| IBIS file stm32n657_vfbga169.ibs
[IBIS ver] 4.2
[File name] stm32n657_vfbga169.ibs
[File Rev] 1.1
[Date] 20-09-2024
[Source] Data Created at STMicroelectronics
[Notes]  File originated from ELDO simulations.
[Disclaimer]  This information is for modeling purpose only and is
   not guaranteed. The information is subject to change without
   notice.
[Copyright] Copyright 2024 STMicroelectronics Inc.
|   Component stm32n657_vfbga169
[Component] stm32n657_vfbga169
[Manufacturer] STMicroelectronics
[Package]
| variable   typ   min   max
R_pkg  0  NA  NA
L_pkg  0  NA  NA
C_pkg  0  NA  NA
[Pin]   signal_name   model_name
A1  PDR_ON  nc
A2  NC  nc
A3  OTG2_HSDM  USB2_HS_IBIS
A4  NC  nc
A5  OTG1_HSDM  USB2_HS_IBIS
A6  OTG1_TXRTUNE  nc
A7  PH1-OSC_OUT  isudq_tt
A8  PC11  io8_tt_i3c
A9  PE11  io8_tt
A10  PE13  io8_tt_i3c
A11  PD7  io8_tt
A12  PD1  io8_tt
A13  VSS  gnd
B1  PC14-OSC32_IN  io8_tt_sw
B2  OTG2_ID  nc
B3  OTG2_HSDP  USB2_HS_IBIS
B4  OTG1_ID  nc
B5  OTG1_HSDP  USB2_HS_IBIS
B6  UCPD1_CC1  nc
B7  PH0-OSC_IN  isudq_tt
B8  PC12  io8_tt
B9  PE14  io8_tt_i3c
B10  PE12  io8_tt
B11  PD10  io8_tt
B12  PD0  io8_tt
B13  PD15  io8_tt_i3c
C1  PC15-OSC32_OUT  io8_tt_sw
C2  VBAT  power
C3  OTG2_TXRTUNE  nc
C4  VDDA18USB  power
C5  VDD33USB  power
C6  UCPD1_CC2  nc
C7  PC9  io8_tt_i3c
C8  PH2  io8_tt
C9  PE5  io8_tt_i3c
C10  PD2  io8_tt
C11  PE7  io8_tt
C12  PD3  io8_tt_i3c
C13  PD14  io8_tt_i3c
D1  V08CAP  nc
D2  PC13  io8_tt_tamp
D3  BOOT0  isudq_tt
D4  PWR_ON  io8_tt
D5  VDDA18AON  nc
D6  PC10  io8_tt_i3c
D7  PC8  io8_tt_i3c
D8  VDDIO4  power
D9  PE15  io8_tt_i3c
D10  PD6  io8_tt
D11  PD12  io8_tt
D12  PE8  io8_tt
D13  PD4  io8_tt_i3c
E1  VDDA18PMU  nc
E2  VSSAPMU  nc
E3  VFBSMPS  nc
E4  NRST  ioreset_tt_v18_1v8
E5  VSSAON  nc
E6  VSS  gnd
E7  VDDCORE  nc
E8  VSS  gnd
E9  VDD  power
E10  PB3  io8_tt
E11  PD8  io8_tt
E12  PE10  io8_tt
E13  PE9  io8_tt
F1  VSSSMPS  nc
F2  VSSSMPS  nc
F3  VSSSMPS  nc
F4  VSSSMPS  nc
F5  VSS  gnd
F6  VDDCORE  nc
F7  VSS  gnd
F8  VDDCORE  nc
F9  VSS  gnd
F10  PE2  io8_tt
F11  PE1  io8_tt
F12  PE0  io8_tt
F13  PD11  io8_tt_i3c
G1  VLXSMPS  nc
G2  VLXSMPS  nc
G3  VLXSMPS  nc
G4  VLXSMPS  nc
G5  VDDCORE  nc
G6  VSS  gnd
G7  VDDCORE  nc
G8  VSS  gnd
G9  VDD  power
G10  PB7  io8_tt
G11  PB6  io8_tt
G12  PB0  io8_tt
G13  PE3  io8_tt
H1  VDDSMPS  nc
H2  VDDSMPS  nc
H3  VDDSMPS  nc
H4  VDDSMPS  nc
H5  VSS  gnd
H6  VDDCORE  nc
H7  VSS  gnd
H8  VDDCORE  nc
H9  VSS  gnd
H10  VDDIO3  power
H11  PN11  io8_tt
H12  PN3  io8_tt
H13  PN1  io8_tt
J1  PF4  io8_tt
J2  PF10  io8_tt
J3  PF5  io8_tt
J4  PF3  io8_tt
J5  VDDA18PLL  nc
J6  VSS  gnd
J7  VDDCORE  nc
J8  VSS  gnd
J9  VDD  power
J10  VDDIO3  power
J11  PN2  io8_tt
J12  PN10  io8_tt
J13  PN0  io8_tt
K1  PF2  io8_tt
K2  PF14  io8_tt
K3  PF15  io8_tt
K4  PF7  io8_tt
K5  VSSA  nc
K6  PG14  io8_tt
K7  PA12  io8_tt
K8  PA2  io8_tt
K9  PG13  io8_tt
K10  PB12  io8_tt_i3c
K11  PN7  io8_tt
K12  PN6  io8_tt
K13  PN9  io8_tt
L1  PF8  io8_tt
L2  PF11  io8_tt
L3  PF12  io8_tt
L4  PF13  io8_tt
L5  VDDA18ADC  nc
L6  VDDCSI  nc
L7  PA11  io8_tt
L8  PA8  io8_tt_i3c
L9  PA1  io8_tt
L10  PB11  io8_tt_i3c
L11  PB5  io8_tt_i3c
L12  PN4  io8_tt
L13  PN5  io8_tt
M1  VREFP  nc
M2  CSI_D1N  DPHY_IBIS_L1
M3  CSI_CKN  DPHY_IBIS_L1
M4  CSI_D0N  DPHY_IBIS_L1
M5  VDDA18CSI  power
M6  PA13  io8_tt
M7  PA9  io8_tt_i3c
M8  PA5  io8_tt_i3c
M9  PA0  io8_tt
M10  PB10  io8_tt_i3c
M11  PB4  io8_tt
M12  PN12  io8_tt
M13  PN8  io8_tt
N1  VSS  gnd
N2  CSI_D1P  DPHY_IBIS_L1
N3  CSI_CKP  DPHY_IBIS_L1
N4  CSI_D0P  DPHY_IBIS_L1
N5  CSI_REXT  nc
N6  PA14  io8_tt
N7  PA10  io8_tt
N8  PA6  io8_tt_i3c
N9  PG10  io8_tt
N10  PG2  io8_tt
N11  PA15  io8_tt
N12  PA3  io8_tt
N13  VSS  gnd
[Package Model]   486-fcvfbga-6x6-169-240308
[Pin Mapping]   pulldown_ref   pullup_ref   | Comment
A1  nc  nc
A2  nc  nc
A3  gnd  VDD33USB
A4  nc  nc
A5  gnd  VDD33USB
A6  nc  nc
A7  gnd  VDD
A8  gnd  VDDIO4
A9  gnd  VDD
A10  gnd  VDD
A11  gnd  VDD
A12  gnd  VDD
A13  gnd  nc
B1  gnd  VSW
B2  nc  nc
B3  gnd  VDD33USB
B4  nc  nc
B5  gnd  VDD33USB
B6  nc  nc
B7  gnd  VDD
B8  gnd  VDDIO4
B9  gnd  VDD
B10  gnd  VDD
B11  gnd  VDD
B12  gnd  VDD
B13  gnd  VDD
C1  gnd  VSW
C2  nc  VSW
C3  nc  nc
C4  nc  VDDA18USB
C5  nc  VDD33USB
C6  nc  nc
C7  gnd  VDDIO4
C8  gnd  VDDIO4
C9  gnd  VDD
C10  gnd  VDD
C11  gnd  VDD
C12  gnd  VDD
C13  gnd  VDD
D1  nc  nc
D2  gnd  VSW
D3  gnd  VDD
D4  gnd  VDD
D5  nc  nc
D6  gnd  VDDIO4
D7  gnd  VDDIO4
D8  nc  VDDIO4
D9  gnd  VDD
D10  gnd  VDD
D11  gnd  VDD
D12  gnd  VDD
D13  gnd  VDD
E1  nc  nc
E2  nc  nc
E3  nc  nc
E4  gnd  VDD
E5  nc  nc
E6  gnd  nc
E7  nc  nc
E8  gnd  nc
E9  nc  VDD
E10  gnd  VDD
E11  gnd  VDD
E12  gnd  VDD
E13  gnd  VDD
F1  nc  nc
F2  nc  nc
F3  nc  nc
F4  nc  nc
F5  gnd  nc
F6  nc  nc
F7  gnd  nc
F8  nc  nc
F9  gnd  nc
F10  gnd  VDD
F11  gnd  VDD
F12  gnd  VDD
F13  gnd  VDD
G1  nc  nc
G2  nc  nc
G3  nc  nc
G4  nc  nc
G5  nc  nc
G6  gnd  nc
G7  nc  nc
G8  gnd  nc
G9  nc  VDD
G10  gnd  VDD
G11  gnd  VDD
G12  gnd  VDD
G13  gnd  VDD
H1  nc  nc
H2  nc  nc
H3  nc  nc
H4  nc  nc
H5  gnd  nc
H6  nc  nc
H7  gnd  nc
H8  nc  nc
H9  gnd  nc
H10  nc  VDDIO3
H11  gnd  VDDIO3
H12  gnd  VDDIO3
H13  gnd  VDDIO3
J1  gnd  VDD
J2  gnd  VDD
J3  gnd  VDD
J4  gnd  VDD
J5  nc  nc
J6  gnd  nc
J7  nc  nc
J8  gnd  nc
J9  nc  VDD
J10  nc  VDDIO3
J11  gnd  VDDIO3
J12  gnd  VDDIO3
J13  gnd  VDDIO3
K1  gnd  VDD
K2  gnd  VDD
K3  gnd  VDD
K4  gnd  VDD
K5  nc  nc
K6  gnd  VDD
K7  gnd  VDD
K8  gnd  VDD
K9  gnd  VDD
K10  gnd  VDD
K11  gnd  VDDIO3
K12  gnd  VDDIO3
K13  gnd  VDDIO3
L1  gnd  VDD
L2  gnd  VDD
L3  gnd  VDD
L4  gnd  VDD
L5  nc  nc
L6  nc  nc
L7  gnd  VDD
L8  gnd  VDD
L9  gnd  VDD
L10  gnd  VDD
L11  gnd  VDD
L12  gnd  VDDIO3
L13  gnd  VDDIO3
M1  nc  nc
M2  gnd  VDDA18CSI
M3  gnd  VDDA18CSI
M4  gnd  VDDA18CSI
M5  nc  VDDA18CSI
M6  gnd  VDD
M7  gnd  VDD
M8  gnd  VDD
M9  gnd  VDD
M10  gnd  VDD
M11  gnd  VDD
M12  gnd  VDDIO3
M13  gnd  VDDIO3
N1  gnd  nc
N2  gnd  VDDA18CSI
N3  gnd  VDDA18CSI
N4  gnd  VDDA18CSI
N5  nc  nc
N6  gnd  VDD
N7  gnd  VDD
N8  gnd  VDD
N9  gnd  VDD
N10  gnd  VDD
N11  gnd  VDD
N12  gnd  VDD
N13  gnd  nc
[Diff Pin]  inv_pin  vdiff  tdelay_typ  tdelay_min  tdelay_max
N3  M3  NA  NA  NA  NA
N4  M4  NA  NA  NA  NA
N2  M2  NA  NA  NA  NA
B5  A5  NA  NA  NA  NA
B3  A3  NA  NA  NA  NA
[Model Selector] DPHY_IBIS_L1
DPHY_RX_2P5G_L1   DPHY HSRX model at 2.5Gbps for lane 1
DPHY_RX_1P5G_L1   DPHY HSRX model at 1.5Gbps for lane 1
[Model Selector] io8_tt
io8_tt_ls_3v3 "GPIO - 3V tolerant - low speed - 3.3V range"
io8_tt_ms_3v3 "GPIO - 3V tolerant - med speed - 3.3V range"
io8_tt_fs_3v3 "GPIO - 3V tolerant - fast speed - 3.3V range"
io8_tt_hs_3v3 "GPIO - 3V tolerant - high speed - 3.3V range"
io8_tt_hslv_ls_1v8 "GPIO low voltage optimization - 3V tolerant - low speed - 1.8V range"
io8_tt_hslv_ms_1v8 "GPIO low voltage optimization - 3V tolerant - med speed - 1.8V range"
io8_tt_hslv_fs_1v8 "GPIO low voltage optimization - 3V tolerant - fast speed - 1.8V range"
io8_tt_hslv_hs_1v8 "GPIO low voltage optimization - 3V tolerant - high speed - 1.8V range"
[Model Selector] io8_tt_i3c
io8_tt_ls_3v3 "GPIO - 3V tolerant - low speed - 3.3V range"
io8_tt_ms_3v3 "GPIO - 3V tolerant - med speed - 3.3V range"
io8_tt_fs_3v3 "GPIO - 3V tolerant - fast speed - 3.3V range"
io8_tt_hs_3v3 "GPIO - 3V tolerant - high speed - 3.3V range"
io8_tt_hslv_ls_1v8 "GPIO low voltage optimization - 3V tolerant - low speed - 1.8V range"
io8_tt_hslv_ms_1v8 "GPIO low voltage optimization - 3V tolerant - med speed - 1.8V range"
io8_tt_hslv_fs_1v8 "GPIO low voltage optimization - 3V tolerant - fast speed - 1.8V range"
io8_tt_hslv_hs_1v8 "GPIO low voltage optimization - 3V tolerant - high speed - 1.8V range"
io8_tt_i3c_ls_3v3 "GPIO with I3C open-drain - 3V tolerant - low speed - 3.3V range"
io8_tt_i3c_ms_3v3 "GPIO with I3C open-drain - 3V tolerant - med speed - 3.3V range"
io8_tt_i3c_fs_3v3 "GPIO with I3C open-drain - 3V tolerant - fast speed - 3.3V range"
io8_tt_i3c_hs_3v3 "GPIO with I3C open-drain - 3V tolerant - high speed - 3.3V range"
io8_tt_hslv_i3c_ls_1v8 "GPIO low voltage optimization with I3C open-drain - 3V tolerant - low speed - 1.8V range"
io8_tt_hslv_i3c_ms_1v8 "GPIO low voltage optimization with I3C open-drain - 3V tolerant - med speed - 1.8V range"
io8_tt_hslv_i3c_fs_1v8 "GPIO low voltage optimization with I3C open-drain - 3V tolerant - fast speed - 1.8V range"
io8_tt_hslv_i3c_hs_1v8 "GPIO low voltage optimization with I3C open-drain - 3V tolerant - high speed - 1.8V range"
io8_tt_i3c_fmp_3v3 "GPIO with I3C fm+ open-drain - 3V tolerant - 3.3V range"
[Model Selector] io8_tt_sw
io8_tt_sw_3v3 "Input Buffer - 3V tolerant - 3.3V range"
io8_tt_sw_1v8 "Input Buffer - 3V tolerant - 1.8V range"
[Model Selector] io8_tt_tamp
io8_tt_ls_3v3 "GPIO - 3V tolerant - low speed - 3.3V range"
io8_tt_ms_3v3 "GPIO - 3V tolerant - med speed - 3.3V range"
io8_tt_fs_3v3 "GPIO - 3V tolerant - fast speed - 3.3V range"
io8_tt_hs_3v3 "GPIO - 3V tolerant - high speed - 3.3V range"
io8_tt_hslv_ls_1v8 "GPIO low voltage optimization - 3V tolerant - low speed - 1.8V range"
io8_tt_hslv_ms_1v8 "GPIO low voltage optimization - 3V tolerant - med speed - 1.8V range"
io8_tt_hslv_fs_1v8 "GPIO low voltage optimization - 3V tolerant - fast speed - 1.8V range"
io8_tt_hslv_hs_1v8 "GPIO low voltage optimization - 3V tolerant - high speed - 1.8V range"
io8_tt_tamp_3v3 "IO tamper - 3V tolerant - 3.3V range"
io8_tt_tamp_1v8 "IO tamper - 3V tolerant - 1.8V range"
|[Model Selector] ioreset_tt_v18
|ioreset_tt_v18_1v8 "Reset PAD - 3V tolerant - 1.8V range"
[Model Selector] isudq_tt
isudq_tt_3v3 "Input Buffer - 3V tolerant - 3.3V range"
isudq_tt_1v8 "Input Buffer - 3V tolerant - 1.8V range"
[Model Selector] USB2_HS_IBIS
USB2_HSRX   USB2 HSRX model
USB2_HSTX_00_0_01_0011_11   TuningBits_AMP_PULSE_RISE_REF_XV=00_0_01_0011_11
USB2_HSTX_00_0_10_0101_11   TuningBits_AMP_PULSE_RISE_REF_XV=00_0_10_0101_11
USB2_HSTX_00_0_11_0111_11   TuningBits_AMP_PULSE_RISE_REF_XV=00_0_11_0111_11
USB2_HSTX_00_1_01_0011_11   TuningBits_AMP_PULSE_RISE_REF_XV=00_1_01_0011_11
USB2_HSTX_00_1_10_0101_11   TuningBits_AMP_PULSE_RISE_REF_XV=00_1_10_0101_11
USB2_HSTX_00_1_11_0111_11   TuningBits_AMP_PULSE_RISE_REF_XV=00_1_11_0111_11
USB2_HSTX_01_0_01_0011_11   TuningBits_AMP_PULSE_RISE_REF_XV=01_0_01_0011_11
USB2_HSTX_01_0_10_0101_11   TuningBits_AMP_PULSE_RISE_REF_XV=01_0_10_0101_11
USB2_HSTX_01_0_11_0111_11   TuningBits_AMP_PULSE_RISE_REF_XV=01_0_11_0111_11
USB2_HSTX_01_1_01_0011_11   TuningBits_AMP_PULSE_RISE_REF_XV=01_1_01_0011_11
USB2_HSTX_01_1_10_0101_11   TuningBits_AMP_PULSE_RISE_REF_XV=01_1_10_0101_11
USB2_HSTX_01_1_11_0111_11   TuningBits_AMP_PULSE_RISE_REF_XV=01_1_11_0111_11
USB2_HSTX_10_0_01_0011_11   TuningBits_AMP_PULSE_RISE_REF_XV=10_0_01_0011_11
USB2_HSTX_10_0_10_0101_11   TuningBits_AMP_PULSE_RISE_REF_XV=10_0_10_0101_11
USB2_HSTX_10_0_11_0111_11   TuningBits_AMP_PULSE_RISE_REF_XV=10_0_11_0111_11
USB2_HSTX_10_1_01_0011_11   TuningBits_AMP_PULSE_RISE_REF_XV=10_1_01_0011_11
USB2_HSTX_10_1_10_0101_11   TuningBits_AMP_PULSE_RISE_REF_XV=10_1_10_0101_11
USB2_HSTX_10_1_11_0111_11   TuningBits_AMP_PULSE_RISE_REF_XV=10_1_11_0111_11
[Define Package Model]  486-fcvfbga-6x6-169-240308
[Manufacturer]  unknown
[OEM]  unknown
[Description]  unknown
[Number Of Pins]  136
[Pin Numbers]
| Pin Name Terminal   Net Name   Starting Node   Ending Node
D3 | BOOT0
M3 | CSI_CKN
N3 | CSI_CKP
M4 | CSI_D0N
N4 | CSI_D0P
M2 | CSI_D1N
N2 | CSI_D1P
N5 | CSI_REXT
E4 | NRST
A5 | OTG1_HSDM
B5 | OTG1_HSDP
B4 | OTG1_ID
A6 | OTG1_TXRTUNE
A4 | NC
A3 | OTG2_HSDM
B3 | OTG2_HSDP
B2 | OTG2_ID
C3 | OTG2_TXRTUNE
A2 | NC
M9 | PA0
L9 | PA1
K8 | PA2
N12 | PA3
M8 | PA5
N8 | PA6
L8 | PA8
M7 | PA9
N7 | PA10
L7 | PA11
K7 | PA12
M6 | PA13
N6 | PA14
N11 | PA15
G12 | PB0
E10 | PB3
M11 | PB4
L11 | PB5
G11 | PB6
G10 | PB7
M10 | PB10
L10 | PB11
K10 | PB12
D7 | PC8
C7 | PC9
D6 | PC10
A8 | PC11
B8 | PC12
D2 | PC13
B1 | PC14-OSC32_IN
C1 | PC15-OSC32_OUT
B12 | PD0
A12 | PD1
C10 | PD2
C12 | PD3
D13 | PD4
D10 | PD6
A11 | PD7
E11 | PD8
B11 | PD10
F13 | PD11
D11 | PD12
C13 | PD14
B13 | PD15
A1 | PDR_ON
F12 | PE0
F11 | PE1
F10 | PE2
G13 | PE3
C9 | PE5
C11 | PE7
D12 | PE8
E13 | PE9
E12 | PE10
A9 | PE11
B10 | PE12
A10 | PE13
B9 | PE14
D9 | PE15
K1 | PF2
J4 | PF3
J1 | PF4
J3 | PF5
K4 | PF7
L1 | PF8
J2 | PF10
L2 | PF11
L3 | PF12
L4 | PF13
K2 | PF14
K3 | PF15
N10 | PG2
N9 | PG10
K9 | PG13
K6 | PG14
B7 | PH0-OSC_IN
A7 | PH1-OSC_OUT
C8 | PH2
J13 | PN0
H13 | PN1
J11 | PN2
H12 | PN3
L12 | PN4
L13 | PN5
K12 | PN6
K11 | PN7
M13 | PN8
K13 | PN9
J12 | PN10
H11 | PN11
M12 | PN12
D4 | PWR_ON
B6 | UCPD1_CC1
C6 | UCPD1_CC2
D1 | V08CAP
C2 | VBAT
C5 | VDD33USB
E9 | VDD
L5 | VDDA18ADC
D5 | VDDA18AON
M5 | VDDA18CSI
J5 | VDDA18PLL
E1 | VDDA18PMU
C4 | VDDA18USB
E7 | VDDCORE
L6 | VDDCSI
H10 | VDDIO3
D8 | VDDIO4
H1 | VDDSMPS
E3 | VFBSMPS
G1 | VLXSMPS
M1 | VREFP
A13 | VSS
K5 | VSSA
E5 | VSSAON
E2 | VSSAPMU
F1 | VSSSMPS
|[Merged Pins]  E9
|G9  |  VDD
|J9  |  VDD
|[Merged Pins]  E7
|F6  |  VDDCORE
|F8  |  VDDCORE
|G5  |  VDDCORE
|G7  |  VDDCORE
|H6  |  VDDCORE
|H8  |  VDDCORE
|J7  |  VDDCORE
|[Merged Pins]  H10
|J10  |  VDDIO3
|[Merged Pins]  H1
|H2  |  VDDSMPS
|H3  |  VDDSMPS
|H4  |  VDDSMPS
|[Merged Pins]  G1
|G2  |  VLXSMPS
|G3  |  VLXSMPS
|G4  |  VLXSMPS
|[Merged Pins]  A13
|E6  |  VSS
|E8  |  VSS
|F5  |  VSS
|F7  |  VSS
|F9  |  VSS
|G6  |  VSS
|G8  |  VSS
|H5  |  VSS
|H7  |  VSS
|H9  |  VSS
|J6  |  VSS
|J8  |  VSS
|N1  |  VSS
|N13  |  VSS
|[Merged Pins]  F1
|F2  |  VSSSMPS
|F3  |  VSSSMPS
|F4  |  VSSSMPS
[Model Data]
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[End Model Data]
[End Package Model]
|End [Component]
| Models and submodels in the file (45): DPHY_RX_1P5G_L1 (Input), DPHY_RX_2P5G_L1 (Input), io8_tt_fs_3v3 (I/O), io8_tt_hs_3v3 (I/O), io8_tt_hslv_fs_1v8 (I/O), io8_tt_hslv_hs_1v8 (I/O), io8_tt_hslv_i3c_fs_1v8 (I/O_open_drain), io8_tt_hslv_i3c_hs_1v8 (I/O_open_drain), io8_tt_hslv_i3c_ls_1v8 (I/O_open_drain), io8_tt_hslv_i3c_ms_1v8 (I/O_open_drain), io8_tt_hslv_ls_1v8 (I/O), io8_tt_hslv_ms_1v8 (I/O), io8_tt_i3c_fmp_3v3 (I/O_open_drain), io8_tt_i3c_fs_3v3 (I/O_open_drain), io8_tt_i3c_hs_3v3 (I/O_open_drain), io8_tt_i3c_ls_3v3 (I/O_open_drain), io8_tt_i3c_ms_3v3 (I/O_open_drain), io8_tt_ls_3v3 (I/O), io8_tt_ms_3v3 (I/O), io8_tt_sw_1v8 (I/O), io8_tt_sw_3v3 (I/O), io8_tt_tamp_1v8 (I/O), io8_tt_tamp_3v3 (I/O), ioreset_tt_v18_1v8 (I/O_open_drain), isudq_tt_1v8 (Input), isudq_tt_3v3 (Input), USB2_HSRX (Input), USB2_HSTX_00_0_01_0011_11 (Output), USB2_HSTX_00_0_10_0101_11 (Output), USB2_HSTX_00_0_11_0111_11 (Output), USB2_HSTX_00_1_01_0011_11 (Output), USB2_HSTX_00_1_10_0101_11 (Output), USB2_HSTX_00_1_11_0111_11 (Output), USB2_HSTX_01_0_01_0011_11 (Output), USB2_HSTX_01_0_10_0101_11 (Output), USB2_HSTX_01_0_11_0111_11 (Output), USB2_HSTX_01_1_01_0011_11 (Output), USB2_HSTX_01_1_10_0101_11 (Output), USB2_HSTX_01_1_11_0111_11 (Output), USB2_HSTX_10_0_01_0011_11 (Output), USB2_HSTX_10_0_10_0101_11 (Output), USB2_HSTX_10_0_11_0111_11 (Output), USB2_HSTX_10_1_01_0011_11 (Output), USB2_HSTX_10_1_10_0101_11 (Output), USB2_HSTX_10_1_11_0111_11 (Output)
